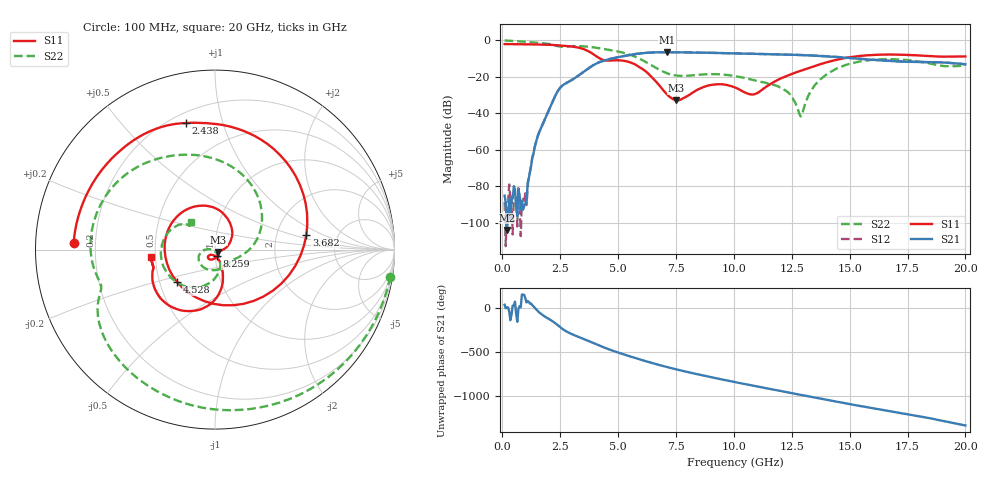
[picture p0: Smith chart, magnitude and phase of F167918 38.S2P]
!  2-Port S-parameters saved by WinCal
! VAR MeasName=S-Parameters (CALIBRATED_DATA) read from VNA (N5242A)
! VAR MeasDate=2016-11-22 10:26:35
! VAR NAME=F167918 38
! VAR FILENAME=F167918 38.S2P
! VAR DATE=2016-11-22 10:26:35
! VAR PHYS_PORTS=1,2
# Hz S DB R 50
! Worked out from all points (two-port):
!   401 points, 100 MHz to 20 GHz, reference 50 ohm
!   highest |S21| = -6.53 dB at 7.115 GHz (marker M1); lowest = -103.9 dB at 199.5 MHz (marker M2)
!   |S21| within 3 dB of the highest: 4.904 GHz to 14.8 GHz (9.901 GHz wide, 100 % of centre)
!   lowest |S11| = -32.9 dB at 7.513 GHz (marker M3), VSWR 1.05, Z = 51.9 - j1.36 ohm
!   |S11| at or under -10 dB: 4.219 GHz to 14.69 GHz (10.48 GHz wide, 111 % of centre)
!   |S22| runs from -41.7 to -0.1 dB; largest |S21 - S12| = 0.0057
!   S11 on the Smith chart (normalised r, x): 100 MHz: 0.12, +0.02; 2.438 GHz: 0.26, +0.77; 3.682 GHz: 2.96, +0.66; 4.528 GHz: 0.62, -0.24; 8.259 GHz: 1.01, -0.08; 20 GHz: 0.47, -0.04
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1e8  -2.07 177.3  -85.12 34.7  -88.70 59.5  -0.10 -8.8
1.995e8  -2.08 174.6  -103.89 3.0  -88.76 -19.1  -0.16 -17.0
1.04525e9  -2.21 151.8  -89.32 60.7  -90.28 128.5  -0.88 -81.1
1.54275e9  -2.32 137.0  -52.08 -39.6  -52.10 -38.6  -1.40 -113.1
2.43825e9  -2.81 102.8  -27.03 153.2  -27.03 152.9  -3.38 -160.0
3.43325e9  -4.51 37.4  -17.98 14.3  -18.00 14.4  -3.26 160.7
3.682e9  -5.76 9.1  -15.69 -12.4  -15.69 -12.2  -3.49 148.7
4.12975e9  -9.33 -62.2  -12.36 -62.7  -12.31 -62.6  -4.23 127.5
4.52775e9  -11.12 -139.3  -10.63 -105.1  -10.58 -105.4  -5.05 109.2
5.62225e9  -12.56 92.1  -7.78 158.4  -7.79 158.0  -8.44 50.8
6.7665e9  -24.51 8.7  -6.57 69.5  -6.59 69.5  -16.05 -10.5
7.11475e9  -29.55 -12.1  -6.53 45.4  -6.55 45.4  -18.09 -23.8
7.51275e9  -32.91 -35.5  -6.55 19.3  -6.57 19.3  -19.29 -39.1
8.259e9  -28.35 -77.3  -6.68 -26.6  -6.68 -26.5  -19.20 -74.4
1.005e10  -25.86 -136.2  -7.16 -126.2  -7.18 -126.1  -19.69 -151.8
1.0846e10  -29.71 -102.4  -7.41 -167.5  -7.40 -167.5  -21.76 -167.5
1.204e10  -20.89 -68.7  -7.77 131.7  -7.75 131.7  -26.02 179.1
1.288575e10  -16.71 -72.3  -8.10 88.7  -8.07 88.9  -41.72 -126.5
1.338325e10  -14.54 -76.6  -8.34 63.6  -8.30 63.9  -26.67 -60.5
1.4627e10  -10.16 -96.1  -9.34 1.6  -9.26 1.5  -14.50 -99.3
1.67165e10  -7.82 -137.3  -11.29 -96.3  -11.25 -96.7  -10.38 -171.3
2e10  -8.84 -173.8  -13.15 100.2  -13.12 99.5  -13.80 131.0
